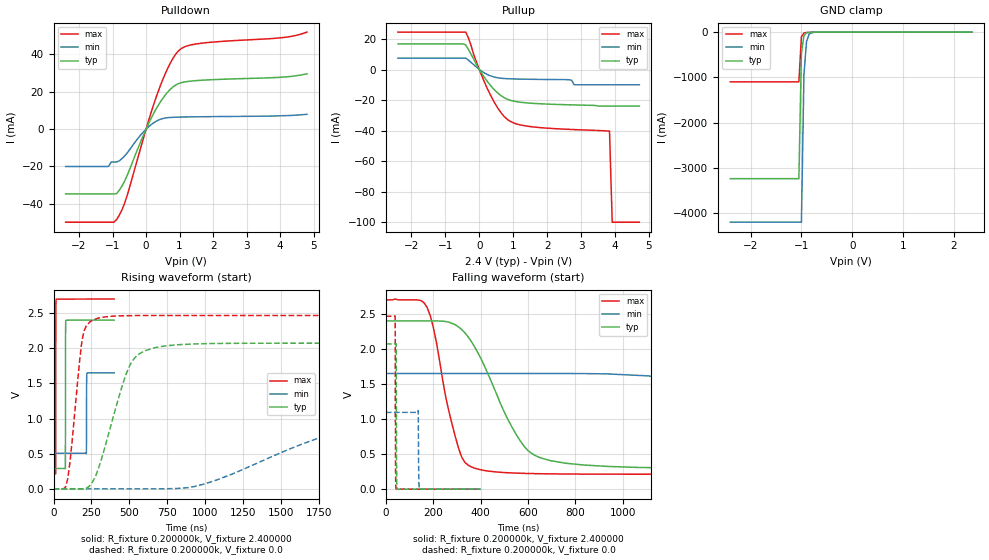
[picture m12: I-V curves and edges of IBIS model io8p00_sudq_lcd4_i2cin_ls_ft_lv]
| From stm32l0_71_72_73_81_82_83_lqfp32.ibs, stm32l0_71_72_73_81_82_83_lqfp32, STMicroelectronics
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|   Model io8p00_sudq_lcd4_i2cin_ls_ft_lv
[Model]  io8p00_sudq_lcd4_i2cin_ls_ft_lv
Model_type I/O
Polarity   Non-Inverting
Enable   Active-Low
Vinl =   0.720000V
Vinh =   1.680000V
Vmeas =  1.200000V
Cref =   50.000000pF
Rref =   100.000000M
Vref =   0.0V
C_comp   2.470900pF   2.435200pF   2.490500pF
[Temperature Range]   25.000000   0.105000k   -40.000000
[Pullup Reference]   2.400000V   1.650000V   2.700000V
[Pulldown Reference]   0.0V   0.0V   0.0V
[POWER Clamp Reference]   2.400000V   1.650000V   2.700000V
[GND Clamp Reference]   0.0V   0.0V   0.0V
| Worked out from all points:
|   slope of the pulldown table from 0 to 0.36 V, typ, clamps not added: 28.5 ohm
|   slope of the pullup table from 0 to 0.36 V, typ, clamps not added: 32.2 ohm
|   GND clamp passes 1 mA (typ) near -0.64 V on its own axis
|   rising waveform, R_fixture 0.200000k, V_fixture 2.400000: 20-80 % time 679ps typ, 856ps min, 745ps max; typ from 0.291 V to 2.4 V
|   rising waveform, R_fixture 0.200000k, V_fixture 0.0: 20-80 % time 169ns typ, 817ns min, 66.4ns max; typ from 0 V to 2.07 V
|   falling waveform, R_fixture 0.200000k, V_fixture 2.400000: 20-80 % time 180ns typ, 726ns min, 89.6ns max; typ from 2.4 V to 0.291 V
|   falling waveform, R_fixture 0.200000k, V_fixture 0.0: 20-80 % time 1.13ns typ, 1.66ns min, 924ps max; typ from 2.07 V to 0 V
[Pulldown]
|Voltage   I(typ)   I(min)   I(max)
-2.4V     -34.7mA    -20mA      -49.82mA
-1.12V    -34.7mA    -20mA      -49.82mA
-1.04V    -34.7mA    -17.6mA    -49.82mA
-880mV    -34.55mA   -17.6mA    -48.46mA
-560mV    -24.65mA   -12.68mA   -35.33mA
0V        326fA      0A         16fA
400mV     13.84mA    5.066mA    22.03mA
720mV     21.24mA    6.254mA    35.26mA
1.04V     24.82mA    6.464mA    43.03mA
1.6V      26.11mA    6.627mA    45.88mA
4V        27.76mA    7.125mA    48.87mA
4.8V      29.63mA    7.94mA     51.96mA
[Pullup]
|Voltage   I(typ)   I(min)   I(max)
-2.4V     16.77mA    7.419mA    24.51mA
-400mV    16.1mA     7.419mA    24.51mA
0V        80fA       7.57pA     0A
320mV     -10.16mA   -4.078mA   -16.34mA
640mV     -17.08mA   -5.718mA   -28.28mA
960mV     -20.45mA   -6.128mA   -34.49mA
1.76V     -22.39mA   -6.47mA    -37.97mA
2.64V     -23.11mA   -6.7mA     -39.19mA
2.8V      -23.2mA    -10mA      -39.35mA
3.84V     -24mA      -10mA      -40.3mA
3.92V     -24mA      -10mA      -100mA
4.72V     -24mA      -10mA      -100mA
[GND_clamp]
|Voltage   I(typ)   I(min)   I(max)
-2.4V     -3.237A    -4.197A    -1.1A
-1.05V    -3.237A    -4.197A    -1.1A
-1V       -475.5mA   -4.197A    -104.1mA
-950mV    -76.08mA   -935.1mA   -18.44mA
-900mV    -16.57mA   -212.6mA   -9.263mA
-850mV    -6.62mA    -50.88mA   -6.764mA
-800mV    -4.092mA   -13.84mA   -4.994mA
-650mV    -1.07mA    -1.21mA    -1.175mA
2.35V     0A         0A         0A
[POWER_clamp]
|Voltage   I(typ)   I(min)   I(max)
-2.4V     0A         0A         0A
0V        0A         0A         0A
[Ramp]
| variable   typ   min   max
dV/dt_r  0.65070/0.30186u   0.18995/0.80860u   1.03800/0.14368u
dV/dt_f  0.75690/0.32136u   0.19674/0.84508u   1.13815/0.15969u
R_load = 50.000000
[Rising Waveform]
R_fixture= 0.200000k
V_fixture= 2.400000
V_fixture_min= 1.650000
V_fixture_max= 2.700000
|time   V(typ)   V(min)   V(max)
0s        290.7mV    507.1mV    212.9mV
14.01ns   290.7mV    507.1mV    220mV
15.22ns   290.7mV    507.1mV    2.438V
17.22ns   290.7mV    507.1mV    2.694V
77.68ns   288.9mV    507.1mV    2.7V
79.28ns   2.082V     507.1mV    2.7V
81.68ns   2.396V     507.1mV    2.7V
216.2ns   2.4V       502.4mV    2.7V
221ns     2.4V       1.646V     2.7V
400ns     2.4V       1.65V      2.7V
[Rising Waveform]
R_fixture= 0.200000k
V_fixture= 0.0
V_fixture_min= 0.0
V_fixture_max= 0.0
|time   V(typ)   V(min)   V(max)
0s        1.73nV     10.46nV    1.321nV
93.43ns   -107.6uV   10.46nV    142.5mV
200.2ns   1.486mV    10.46nV    2.239V
280.3ns   198.2mV    -23.36uV   2.418V
373.7ns   864.4mV    -23.46uV   2.454V
547.2ns   1.888V     17.59uV    2.465V
934.3ns   2.062V     36.46mV    2.467V
1.895us   2.072V     817.9mV    2.467V
2.683us   2.072V     1.051V     2.467V
13.33us   2.072V     1.095V     2.467V
[Falling Waveform]
R_fixture= 0.200000k
V_fixture= 2.400000
V_fixture_min= 1.650000
V_fixture_max= 2.700000
|time   V(typ)   V(min)   V(max)
0s        2.4V       1.65V      2.7V
173.5ns   2.4V       1.65V      2.597V
320.3ns   2.276V     1.65V      456.7mV
520.5ns   960.1mV    1.65V      233.2mV
627.3ns   485.6mV    1.65V      222mV
827.5ns   346.9mV    1.649V     215.1mV
1.348us   297.1mV    1.497V     212.9mV
2.162us   291mV      740.8mV    212.9mV
2.789us   290.8mV    568.1mV    212.9mV
13.33us   290.7mV    507.1mV    212.9mV
[Falling Waveform]
R_fixture= 0.200000k
V_fixture= 0.0
V_fixture_min= 0.0
V_fixture_max= 0.0
|time   V(typ)   V(min)   V(max)
0s        2.072V     1.095V     2.467V
39.24ns   2.072V     1.095V     2.471V
40.84ns   2.072V     1.095V     354.6mV
43.64ns   2.07V      1.095V     4.932mV
45.25ns   340.8mV    1.095V     1.411mV
48.05ns   5.265mV    1.095V     498.6uV
136.5ns   25.61uV    1.121V     140.2uV
138.9ns   25.58uV    199.8mV    140.4uV
142.9ns   25.52uV    2.959mV    140.8uV
400ns     1.73nV     10.46nV    1.321nV
